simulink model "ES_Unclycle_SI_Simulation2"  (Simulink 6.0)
settings: Solver=ode45  StartTime=0.0  StopTime=tmax  FixedStep=deltaT  MaxStep=deltaT+.001  MinStep=deltaT-.001  RelTol=1e-3
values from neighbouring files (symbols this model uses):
  ax = .05    (= 0.05)    [ES_Unicycle_Values_SI.m]    (also in ES_PointMass_Values.m; ES_SimplifyPointMass_Values.m; ES_Unstable_Values.m; doublepointmass.m)
  centx = 0    [ES_Unicycle_nc_values_tune_V.m]    (also in ES_Unicycle_nc_values_tune_V_moving.m; ES_Unicycle_Values.m; ES_Unicycle_Values_SI.m = -1; ES_PointMass_Values.m = -1)
  centy = 0    [ES_Unicycle_nc_values_tune_V.m]    (also in ES_Unicycle_nc_values_tune_V_moving.m; ES_Unicycle_Values.m; ES_Unicycle_Values_SI.m = -1; ES_PointMass_Values.m = -1)
  cx = 20    [ES_Unicycle_Values.m]    (also in ES_Unicycle_Values_SI.m = 10; ES_PointMass_Values.m; ES_SimplifyPointMass_Values.m = 15; ES_Unstable_Values.m = 15)
  ICx = 2 - r    (= 1.8)    [ES_Unicycle_nc_values_tune_V.m]    (also in ES_Unicycle_nc_values_tune_V_moving.m = 1.5; ES_Unicycle_Values.m = 2; ES_Unicycle_Values_SI.m = 1; ES_PointMass_Values.m = 1)
  ICy = 2    [ES_Unicycle_nc_values_tune_V.m]    (also in ES_Unicycle_nc_values_tune_V_moving.m; ES_Unicycle_Values.m = 1; ES_Unicycle_Values_SI.m = 1; ES_PointMass_Values.m = 1)
  p1 = 1    [ES_Unicycle_Values_SI.m]    (also in doublepointmass.m; pointmass.m)
  p2 = 1/2    (= 0.5)    [ES_Unicycle_Values_SI.m]    (also in doublepointmass.m; pointmass.m)
  root = 1    [ES_Unicycle_Values_SI.m]    (also in ES_PointMass_Values.m; ES_SimplifyPointMass_Values.m; ES_Unstable_Values.m; doublepointmass.m)
  tmax = 50    [ES_Unicycle_nc_values_tune_V.m]    (also in ES_Unicycle_nc_values_tune_V_moving.m = 300; ES_Unicycle_Values.m = 25; ES_Unicycle_Values_SI.m = 150; ES_PointMass_Values.m)
  wo = wx    (= 20)    [ES_Unicycle_Values_SI.m]
  wx = 20    [ES_Unicycle_Values_SI.m]    (also in ES_PointMass_Values.m = 30; ES_SimplifyPointMass_Values.m = 30; ES_Unstable_Values.m = 30; doublepointmass.m = 30)
undefined symbols (not defined in the file or in its folder): Graph, sfunxy, simulink3, Sinks, XY
libraries: simulink x1

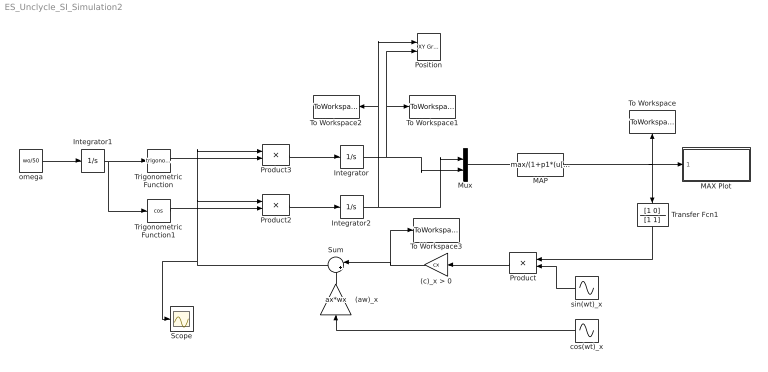
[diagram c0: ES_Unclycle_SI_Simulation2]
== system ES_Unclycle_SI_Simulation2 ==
  (aw)_x : Gain  Orientation=up  Gain=ax*wx
  (c)_x > 0 : Gain  Orientation=left  Gain=cx
  Integrator : Integrator  InitialCondition=ICy
  Integrator1 : Integrator
  Integrator2 : Integrator  InitialCondition=ICx
  MAP : Fcn  Expr=max/(1+p1*(u[1]-centx)^2+p2*(u[2]-centy)^2)^(root)
  MAX Plot : Subsystem
  Mux : Mux  Inputs=2
  Position : simulink/Sinks/XY Graph  xmin=centx - abs(ICx) -1  xmax=centx + abs(ICx) + 2  ymin=centy - abs(ICy)-1  ymax=centy + abs(ICy) + 2  st=-1
  Product : Product  Orientation=left
  Product2 : Product
  Product3 : Product
  Scope : Scope
  Sum : Sum  Orientation=left  Inputs=|++
  To Workspace : ToWorkspace  VariableName=MAX  SampleTime=-1  SaveFormat=Array
  To Workspace1 : ToWorkspace  VariableName=Y  SampleTime=-1  SaveFormat=Array
  To Workspace2 : ToWorkspace  VariableName=X  SampleTime=-1  SaveFormat=Array
  To Workspace3 : ToWorkspace  VariableName=Vx  SampleTime=-1  SaveFormat=Array
  Transfer Fcn1 : TransferFcn  Orientation=down  Numerator=[1 0]  Denominator=[1 1]
  Trigonometric Function : Trigonometry
  Trigonometric Function1 : Trigonometry  Operator=cos
  cos(wt)_x : Sin  Orientation=left  Frequency=wx  Phase=pi/2  SampleTime=0
  omega : Constant  Value=wo/50
  sin(wt)_x : Sin  Orientation=left  Frequency=wx  SampleTime=0
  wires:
  Integrator/1 -> To Workspace1/1, Position/2, Mux/2
  Integrator2/1 -> Mux/1, To Workspace2/1, Position/1
  (aw)_x/1 -> Sum/2
  sin(wt)_x/1 -> Product/2
  (c)_x > 0/1 -> Sum/1, To Workspace3/1
  cos(wt)_x/1 -> (aw)_x/1
  Product/1 -> (c)_x > 0/1
  Mux/1 -> MAP/1
  MAP/1 -> MAX Plot/1(MAX Seeking Value), To Workspace/1, Transfer Fcn1/1
  Transfer Fcn1/1 -> Product/1
  omega/1 -> Integrator1/1
  Product3/1 -> Integrator/1
  Product2/1 -> Integrator2/1
  Trigonometric Function1/1 -> Product2/2
  Trigonometric Function/1 -> Product3/2
  Sum/1 -> Product3/1, Product2/1, Scope/1
  Integrator1/1 -> Trigonometric Function/1, Trigonometric Function1/1

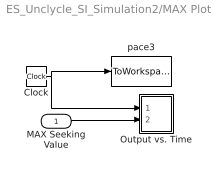
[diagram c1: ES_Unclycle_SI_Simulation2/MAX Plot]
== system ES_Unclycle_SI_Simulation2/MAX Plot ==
  MAX Seeking Value : Inport  Port=1  LatchInput=off
  Clock : Clock
  Output vs. Time : Subsystem  AncestorBlock=simulink3/Sinks/XY Graph  LoadFcn=sfunxy([],[],[],'LoadBlock')  StartFcn=sfunxy([],[],[],'Start')  StopFcn=sfunxy([],[],[],'Stop')  TreatAsAtomicUnit=on  SimViewingDevice=on  mask(XY scope.){xmin=0, xmax=tmax, ymin=-3, ymax=max + 2, st=-1}
      mask prompts: xmin "x-min:"; xmax "x-max:"; ymin "y-min:"; ymax "y-max:"; st "Sample time:"
      mask help: XY scope using MATLAB graph window. First input is used as time base. Enter plotting ranges.
  pace3 : ToWorkspace  VariableName=T  SampleTime=-1  SaveFormat=Array
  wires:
  Clock/1 -> pace3/1, Output vs. Time/1(time)
  MAX Seeking Value/1 -> Output vs. Time/2(MAX Seeking Value)

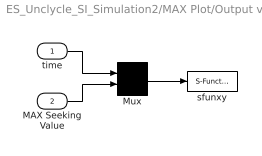
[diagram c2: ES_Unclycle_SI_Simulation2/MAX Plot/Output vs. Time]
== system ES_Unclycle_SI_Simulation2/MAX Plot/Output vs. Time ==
  time : Inport  Port=1  LatchInput=off
  MAX Seeking Value : Inport  Port=2  LatchInput=off
  Mux : Mux  Inputs=2
  sfunxy : S-Function  FunctionName=sfunxy  Parameters=[xmin xmax ymin ymax], st
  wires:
  Mux/1 -> sfunxy/1
  time/1 -> Mux/1
  MAX Seeking Value/1 -> Mux/2
